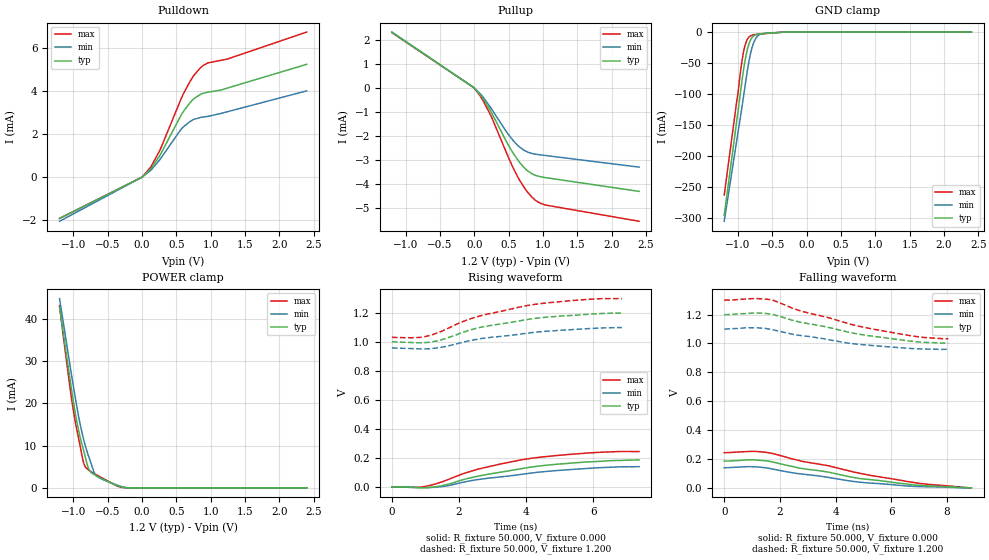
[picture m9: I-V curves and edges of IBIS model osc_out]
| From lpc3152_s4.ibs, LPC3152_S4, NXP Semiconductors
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[Model] osc_out
Model_type Output
Vref=0.000E+00
Rref=1.000E+06
Cref=1.500E-12
Vmeas=9.000E-01
C_comp   9.120E-13   9.060E-13   9.180E-13
[Voltage Range]   1.200E+00   1.100E+00   1.300E+00
[POWER Clamp Reference]   1.200E+00   1.100E+00   1.300E+00
[GND Clamp Reference]   0.000E+00   0.000E+00   0.000E+00
[Pullup Reference]   1.200E+00   1.100E+00   1.300E+00
[Pulldown Reference]   0.000E+00   0.000E+00   0.000E+00
[Temperature Range]   25   85   -40
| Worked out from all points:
|   slope of the pulldown table from 0 to 0.18 V, typ, clamps not added: 287 ohm
|   slope of the pullup table from 0 to 0.18 V, typ, clamps not added: 264 ohm
|   GND clamp passes 1 mA (typ) near -0.45 V on its own axis
|   POWER clamp passes 1 mA (typ) near -0.43 V on its own axis
|   rising waveform, R_fixture 50.000, V_fixture 0.000: 20-80 % time 2.63ns typ, 2.81ns min, 2.43ns max; typ from 0 V to 0.186 V
|   falling waveform, R_fixture 50.000, V_fixture 0.000: 20-80 % time 3.65ns typ, 3.4ns min, 3.88ns max; typ from 0.186 V to 0 V
|   rising waveform, R_fixture 50.000, V_fixture 1.200: 20-80 % time 2.35ns typ, 2.52ns min, 2.32ns max; typ from 1 V to 1.2 V
|   falling waveform, R_fixture 50.000, V_fixture 1.200: 20-80 % time 3.24ns typ, 2.96ns min, 3.3ns max; typ from 1.2 V to 1 V
[GND Clamp]
-1.2V     -295.1mA   -304.5mA   -262.3mA
-1.02V    -144.7mA   -176.3mA   -113.1mA
-1V       -128.4mA   -161.7mA   -98.78mA
-960mV    -94.04mA   -133.9mA   -60.87mA
-920mV    -61.72mA   -104.6mA   -32.69mA
-900mV    -47.82mA   -89.48mA   -22.86mA
-860mV    -26.62mA   -60.2mA    -11mA
-800mV    -9.583mA   -26.93mA   -5.298mA
-760mV    -5.297mA   -14.28mA   -4.232mA
-700mV    -3.225mA   -5.186mA   -3.416mA
-260mV    0A         0A         0A
2.4V      0A         0A         0A
[Power Clamp]
-1.2V     42.74mA    44.8mA     43.16mA
-1.14V    36.05mA    38.59mA    35.19mA
-1.02V    22.7mA     26.17mA    20.5mA
-940mV    14.95mA    18.48mA    13.09mA
-860mV    9.469mA    12.16mA    6.573mA
-820mV    6.968mA    9.666mA    4.847mA
-780mV    4.594mA    7.61mA     4.274mA
-700mV    3.175mA    3.782mA    3.425mA
-660mV    2.803mA    2.765mA    3.062mA
-380mV    646uA      766.2uA    578.3uA
-260mV    67.09uA    138.1uA    34.9uA
2.4V      0A         0A         0A
[Pullup]
-1.2V     2.32mA     2.313mA    2.296mA
0V        0A         0A         0A
100mV     -331uA     -280.1uA   -391.2uA
240mV     -969uA     -823.2uA   -1.147mA
460mV     -2.184mA   -1.787mA   -2.631mA
580mV     -2.765mA   -2.23mA    -3.402mA
660mV     -3.091mA   -2.456mA   -3.83mA
760mV     -3.401mA   -2.641mA   -4.268mA
840mV     -3.564mA   -2.721mA   -4.535mA
900mV     -3.64mA    -2.755mA   -4.683mA
1.04V     -3.725mA   -2.806mA   -4.864mA
2.4V      -4.295mA   -3.288mA   -5.536mA
[Pulldown]
-1.2V     -1.913mA   -2.043mA   -1.911mA
0V        0A         0A         0A
120mV     358uA      295.6uA    437.2uA
260mV     1.004mA    811.7uA    1.242mA
560mV     2.819mA    2.18mA     3.555mA
600mV     3.031mA    2.323mA    3.843mA
740mV     3.589mA    2.654mA    4.643mA
880mV     3.879mA    2.785mA    5.155mA
960mV     3.941mA    2.819mA    5.3mA
1.14V     4.031mA    2.948mA    5.412mA
1.24V     4.128mA    3.032mA    5.472mA
2.4V      5.234mA    4.003mA    6.729mA
[Rising Waveform]
R_fixture = 50.000
V_fixture = 0.000
V_fixture_min = 0.000
V_fixture_max = 0.000
|  time   V(typ)   V(min)   V(max)
0s        0V         0V         0V
710ps     -5.454mV   -3.707mV   -3.648mV
1.06ns    -5.394mV   -5.875mV   5.491mV
1.48ns    6.599mV    1.419mV    33.28mV
2.14ns    50.63mV    32.28mV    91.65mV
2.55ns    72.67mV    49.84mV    120.9mV
4.14ns    135.9mV    94.65mV    196.9mV
5.01ns    157.9mV    113.8mV    218.2mV
6ns       173.6mV    129.7mV    235.9mV
7.36ns    185.6mV    138.9mV    243.6mV
[Falling Waveform]
R_fixture = 50.000
V_fixture = 0.000
V_fixture_min = 0.000
V_fixture_max = 0.000
|  time   V(typ)   V(min)   V(max)
0s        185.6mV    138.9mV    243.6mV
920ps     193.6mV    146.7mV    252mV
1.11ns    192.8mV    145.5mV    252.4mV
1.49ns    187.2mV    138.4mV    245.9mV
1.79ns    176.7mV    128.1mV    235.4mV
2.72ns    135.9mV    97.21mV    187.6mV
3.73ns    109.2mV    72.42mV    153mV
4.86ns    64.49mV    38.99mV    101.1mV
7.04ns    17.15mV    8.179mV    30.21mV
8.88ns    0V         0V         0V
[Rising Waveform]
R_fixture = 50.000
V_fixture = 1.200
V_fixture_min = 1.100
V_fixture_max = 1.300
|  time   V(typ)   V(min)   V(max)
0s        1.002V     959.1mV    1.033V
550ps     997.1mV    955.2mV    1.029V
1.02ns    996.7mV    953.1mV    1.039V
1.47ns    1.015V     963.7mV    1.073V
2.01ns    1.058V     992.4mV    1.132V
2.5ns     1.094V     1.017V     1.173V
4.05ns    1.156V     1.062V     1.253V
4.65ns    1.173V     1.075V     1.271V
5.74ns    1.19V      1.091V     1.293V
6.85ns    1.2V       1.1V       1.3V
[Falling Waveform]
R_fixture = 50.000
V_fixture = 1.200
V_fixture_min = 1.100
V_fixture_max = 1.300
|  time   V(typ)   V(min)   V(max)
0s        1.2V       1.1V       1.3V
820ps     1.208V     1.109V     1.309V
1.61ns    1.205V     1.1V       1.305V
1.88ns    1.194V     1.089V     1.291V
2.78ns    1.145V     1.054V     1.223V
3.55ns    1.12V      1.034V     1.188V
4.42ns    1.08V      1.003V     1.14V
4.92ns    1.062V     992.6mV    1.116V
6.83ns    1.013V     964.1mV    1.05V
8.05ns    1.002V     959.1mV    1.033V
[Ramp]
dV/dt_r   1.1053E-01/2.6381E-09   8.2232E-02/2.8041E-09   1.4522E-01/2.4269E-09
dV/dt_f   1.1454E-01/3.2481E-09   8.0908E-02/2.9713E-09   1.5579E-01/3.2925E-09
R_load = 50
